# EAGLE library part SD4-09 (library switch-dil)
DIL/CODE SWITCH
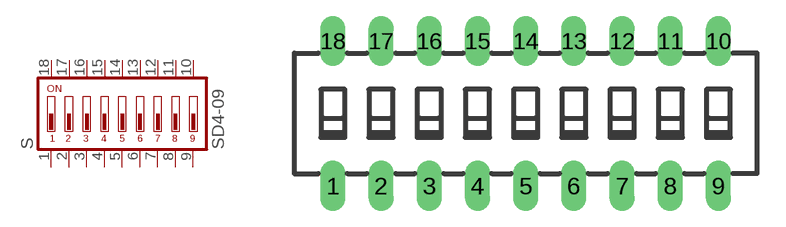
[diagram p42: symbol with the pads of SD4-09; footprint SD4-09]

Designator prefix S

## SD4-09 (OC_FARNELL: unknown; OC_NEWARK: unknown)  [SD4-09]
1  1  pas
2  2  pas
3  3  pas
4  4  pas
5  5  pas
6  6  pas
7  7  pas
8  8  pas
9  9  pas
10  10  pas
11  11  pas
12  12  pas
13  13  pas
14  14  pas
15  15  pas
16  16  pas
17  17  pas
18  18  pas

## Footprint SD4-09 (pad centres in mm)
DIL/CODE SWITCH Mors
drill 0.813 long: 1 -10.16,-3.81; 2 -7.62,-3.81; 3 -5.08,-3.81; 4 -2.54,-3.81; 5 0,-3.81; 6 2.54,-3.81; 7 5.08,-3.81; 8 7.62,-3.81; 9 10.16,-3.81; 10 10.16,3.81; 11 7.62,3.81; 12 5.08,3.81; 13 2.54,3.81; 14 0,3.81; 15 -2.54,3.81; 16 -5.08,3.81; 17 -7.62,3.81; 18 -10.16,3.81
